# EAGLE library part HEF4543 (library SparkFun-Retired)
BCD to 7-seg decoder/driver Not in catalog
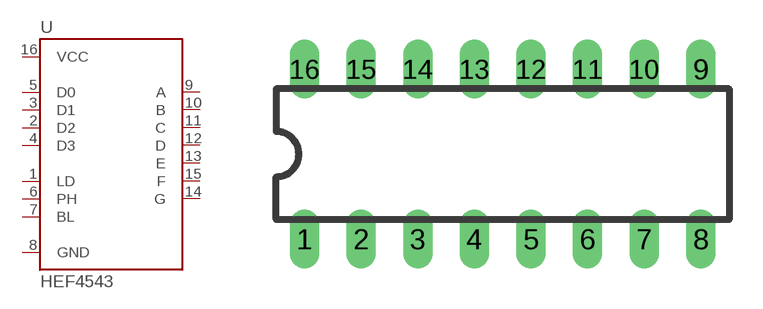
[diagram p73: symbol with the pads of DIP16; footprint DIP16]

Designator prefix -

## HEF4543PTH  [DIP16]
1  LD
2  D2
3  D1
4  D3
5  D0
6  PH
7  BL
8  GND
9  A
10  B
11  C
12  D
13  E
14  G
15  F
16  VCC

## Footprint DIP16 (pad centres in mm)
Dual In Line Package
drill 0.813 long: 1 -8.89,-3.81; 2 -6.35,-3.81; 3 -3.81,-3.81; 4 -1.27,-3.81; 5 1.27,-3.81; 6 3.81,-3.81; 7 6.35,-3.81; 8 8.89,-3.81; 9 8.89,3.81; 10 6.35,3.81; 11 3.81,3.81; 12 1.27,3.81; 13 -1.27,3.81; 14 -3.81,3.81; 15 -6.35,3.81; 16 -8.89,3.81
